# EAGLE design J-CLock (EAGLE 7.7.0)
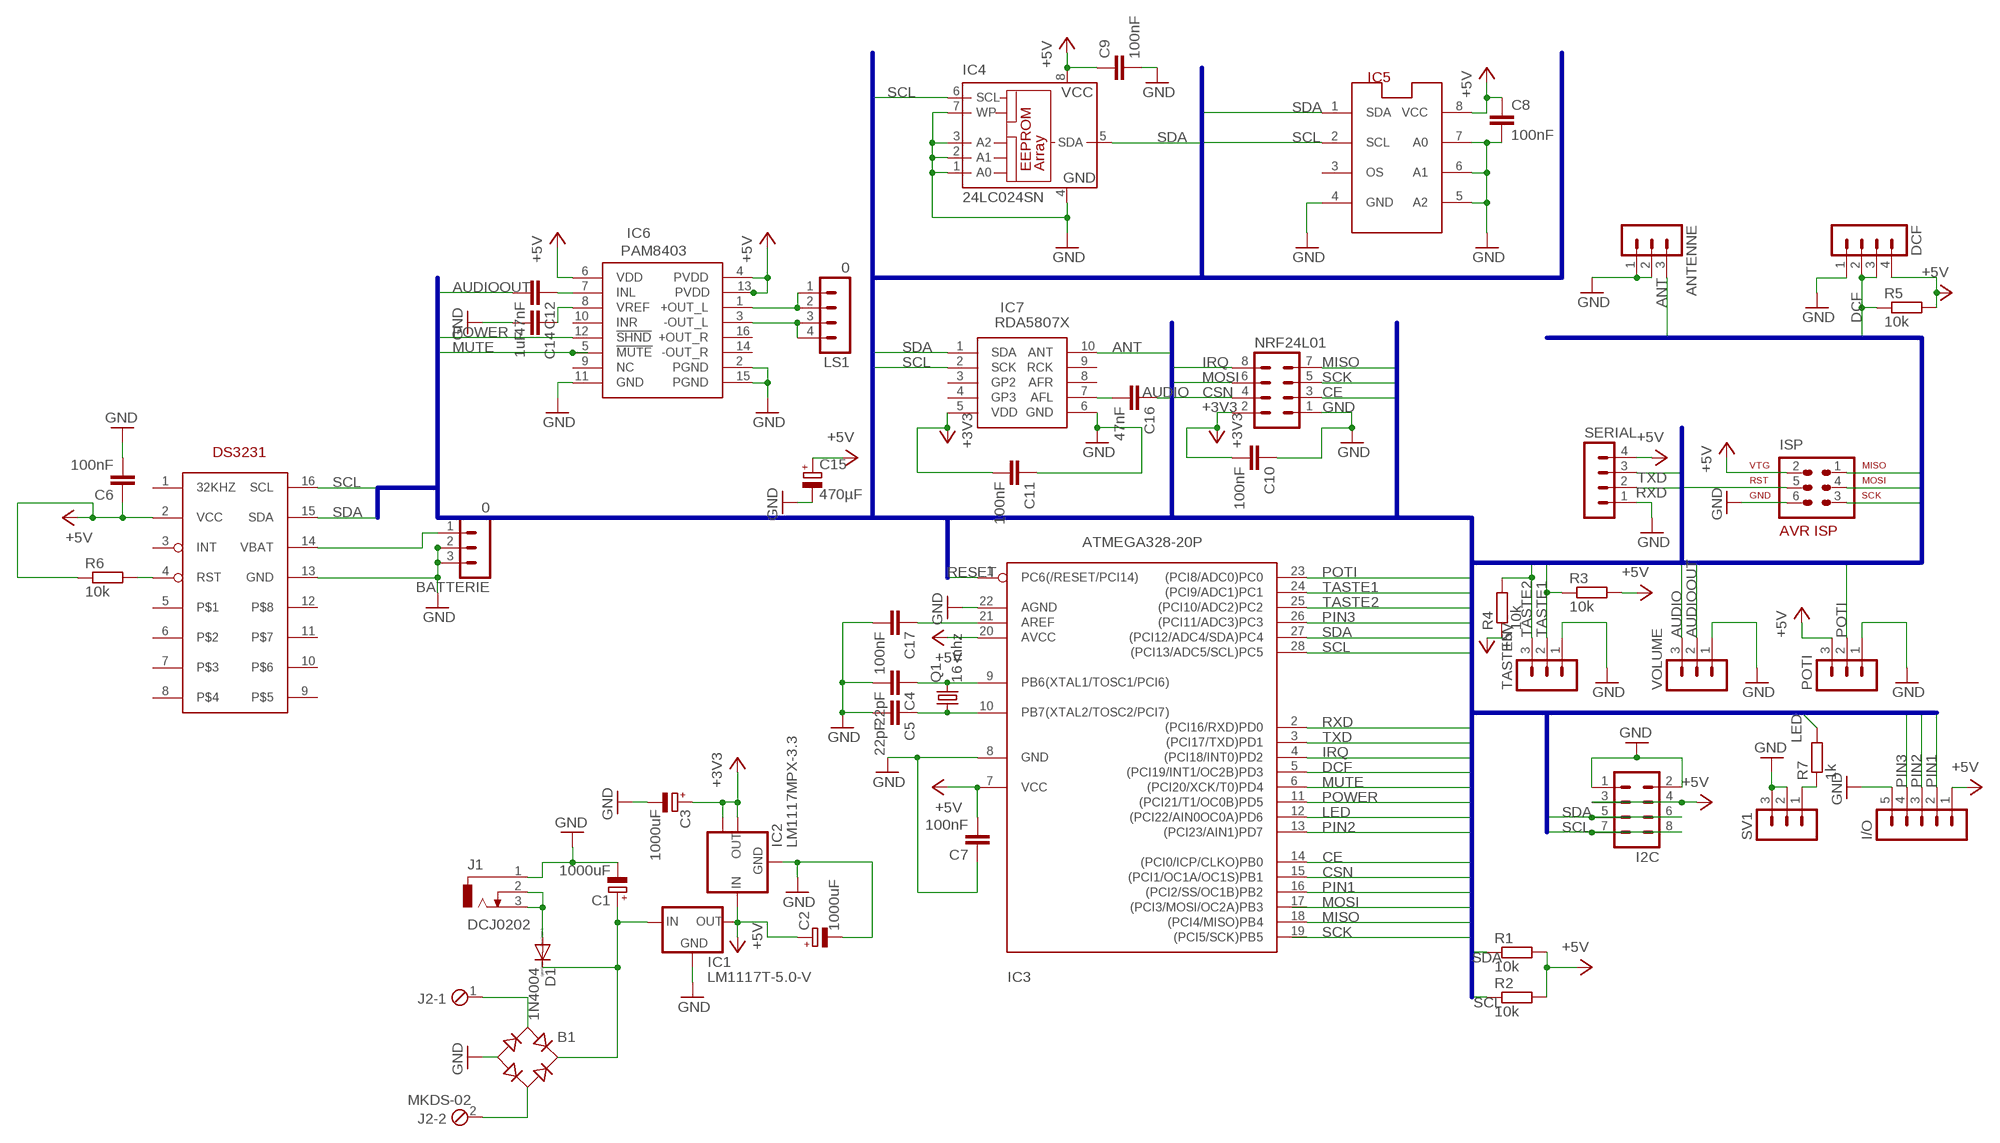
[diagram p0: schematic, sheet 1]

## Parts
ANTENNE  MA03-1  [MA03-1]
B1  B-DIL  [B-DIL]
BATTERIE  0  MA03-1  [MA03-1]
C1  1000uF  CPOL-EUE5-10.5  [E5-10,5]
C2  1000uF  CPOL-EUE5-10.5  [E5-10,5]
C3  1000uF  CPOL-EUE5-10.5  [E5-10,5]
C4  22pF  C-EU050-030X075  [C050-030X075]
C5  22pF  C-EU050-030X075  [C050-030X075]
C6  100nF  C-EU050-030X075  [C050-030X075]
C7  100nF  C-EU050-030X075  [C050-030X075]
C8  100nF  C-EU050-030X075  [C050-030X075]
C9  100nF  C-EU050-030X075  [C050-030X075]
C10  100nF  C-EU050-030X075  [C050-030X075]
C11  100nF  C-EU050-030X075  [C050-030X075]
C12  47nF  C-EU050-030X075  [C050-030X075]
C14  1uF  C-EU050-030X075  [C050-030X075]
C15  470µF  CPOL-EUE3.5-8  [E3,5-8]
C16  47nF  C-EU050-030X075  [C050-030X075]
C17  100nF  C-EU050-030X075  [C050-030X075]
D1  1N4004  [DO41-10]
DCF  MA04-1  [MA04-1]
I2C  MA04-2  [MA04-2]
I/O  MA05-1  [MA05-1]
IC1  LM1117T-5.0-V  [TO220V]
IC2  LM1117MPX-3.3  [SOT223]
IC3  ATMEGA328-20P  [DIL28-3]
IC4  24LC024SN  [SO-08]
IC5  LM75_ICN  [SO8_LM75]
IC6  PAM8403  [SOP16]
IC7  RDA5807X  [MOD5807]
ISP  AVR-ISP-6  [AVR-ISP-6]
J1  DCJ0202  [DCJ0202]
J2  MKDS-02  [MKDS-02]
LS1  0  MA04-1  [MA04-1]
NRF24L01  MA04-2  [MA04-2]
POTI  MA03-1  [MA03-1]
Q1  16 mhz  CRYSTALHC49S  [HC49/S]
R1  10k  R-EU_0207/5V  [0207/5V]
R2  10k  R-EU_0207/5V  [0207/5V]
R3  10k  R-EU_0207/5V  [0207/5V]
R4  10k  R-EU_0207/5V  [0207/5V]
R5  10k  R-EU_0207/5V  [0207/5V]
R6  10k  R-EU_0207/5V  [0207/5V]
R7  1k  R-EU_0207/5V  [0207/5V]
SERIAL  MA04-1  [MA04-1]
SV1  MA03-1  [MA03-1]
TASTEN  MA03-1  [MA03-1]
U$2  DS3231  [SO16]
VOLUME  MA03-1  [MA03-1]

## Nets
+3V3: C3.+ C10.2 C11.2 IC2.2(OUT) IC2.TAB(OUT1) IC7.5(VDD) NRF24L01.2
+5V: C2.+ C6.1 C7.2 C8.1 C9.1 C15.+ DCF.4 I2C.3 I2C.4 I/O.1 IC1.2(OUT) IC2.3(IN) IC3.7(VCC) IC3.20(AVCC) IC4.8(VCC) IC5.8(VCC) IC6.4(PVDD) IC6.6(VDD) IC6.13(PVDD) ISP.2 POTI.3 R1.2 R2.2 R3.2 R4.1 R5.2 R6.1 SERIAL.4 U$2.2(VCC)
ANT: ANTENNE.3 IC7.10(ANT)
AUDIO: C16.1 VOLUME.3
AUDIOOUT: C12.2 VOLUME.2
CE: IC3.14((PCI0/ICP/CLKO)PB0) NRF24L01.3
CSN: IC3.15((PCI1/OC1A/OC1S)PB1) NRF24L01.4
DCF: DCF.2 DCF.3 IC3.5((PCI19/INT1/OC2B)PD3) R5.1
GND: ANTENNE.1 ANTENNE.2 B1.- BATTERIE.2 BATTERIE.3 C1.- C2.- C3.- C4.2 C5.2 C6.2 C7.1 C8.2 C9.2 C10.1 C11.1 C14.2 C15.- C17.2 DCF.1 I2C.1 I2C.2 I/O.5 IC1.1(GND) IC2.1(GND) IC3.8(GND) IC3.22(AGND) IC4.1(A0) IC4.2(A1) IC4.3(A2) IC4.4(GND) IC4.7(WP) IC5.4(GND) IC5.5(A2) IC5.6(A1) IC5.7(A0) IC6.2(PGND) IC6.11(GND) IC6.15(PGND) IC7.6(GND) ISP.6 J1.1 NRF24L01.1 POTI.1 SERIAL.1 SV1.2 SV1.3 TASTEN.1 U$2.13(GND) VOLUME.1
IRQ: IC3.4((PCI18/INT0)PD2) NRF24L01.8
LED: IC3.12((PCI22/AIN0OC0A)PD6) R7.2
MISO: IC3.18((PCI4/MISO)PB4) ISP.1 NRF24L01.7
MOSI: ISP.4 NRF24L01.6
MUTE: IC3.6((PCI20/XCK/T0)PD4) IC6.5(!MUTE!)
N$1: B1.AC2 J2.2
N$2: C4.1 IC3.9(PB6(XTAL1/TOSC1/PCI6)) Q1.2
N$3: B1.+ C1.+ D1.C IC1.3(IN)
N$4: C5.1 IC3.10(PB7(XTAL2/TOSC2/PCI7)) Q1.1
N$5: BATTERIE.1 U$2.14(VBAT)
N$6: D1.A J1.2 J1.3
N$7: B1.AC1 J2.1
N$8: R6.2 U$2.4(RST)
N$9: IC6.1(+OUT_L) LS1.1 LS1.2
N$11: C16.2 IC7.7(AFL)
N$12: C17.1 IC3.21(AREF)
N$14: R7.1 SV1.1
N$16: IC6.3(-OUT_L) LS1.3 LS1.4
N$17: C12.1 IC6.7(INL)
N$18: C14.1 IC6.8(VREF)
PIN1: I/O.2 IC3.16((PCI2/SS/OC1B)PB2)
PIN2: I/O.3 IC3.13((PCI23/AIN1)PD7)
PIN3: I/O.4 IC3.26((PCI11/ADC3)PC3)
POTI: IC3.23((PCI8/ADC0)PC0) POTI.2
POWER: IC3.11((PCI21/T1/OC0B)PD5) IC6.12(!SHND!)
RESET: IC3.1(PC6(/RESET/PCI14)) ISP.5
RXD: IC3.2((PCI16/RXD)PD0) SERIAL.2
SCK: ISP.3 NRF24L01.5
SCL: I2C.7 I2C.8 IC3.28((PCI13/ADC5/SCL)PC5) IC4.6(SCL) IC5.2(SCL) IC7.2(SCK) R2.1 U$2.16(SCL)
SDA: I2C.5 I2C.6 IC3.27((PCI12/ADC4/SDA)PC4) IC4.5(SDA) IC5.1(SDA) IC7.1(SDA) R1.1 U$2.15(SDA)
TASTE1: IC3.24((PCI9/ADC1)PC1) R3.1 TASTEN.2
TASTE2: IC3.25((PCI10/ADC2)PC2) R4.2 TASTEN.3
TXD: IC3.3((PCI17/TXD)PD1) SERIAL.3
Unconnected: IC3.17((PCI3/MOSI/OC2A)PB3) IC3.19((PCI5/SCK)PB5) IC5.3(OS) IC6.9(NC) IC6.10(INR) IC6.14(-OUT_R) IC6.16(+OUT_R) IC7.3(GP2) IC7.4(GP3) IC7.8(AFR) IC7.9(RCK) U$2.1(32KHZ) U$2.3(INT) U$2.5 U$2.6 U$2.7 U$2.8 U$2.9 U$2.10 U$2.11 U$2.12

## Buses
CE,CSN,SCK,MOSI,MISO,IRQ,RESET,SDA,SCL,TXD,RXD,TASTE1,TASTE2,POTI,DCF,MUTE,POWER,LED,AUDIO,AUDIOOUT,LS+,LS-,ANT,PIN1,PIN2,PIN3

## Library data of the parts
ANTENNE BATTERIE POTI SV1 TASTEN VOLUME = con-lstb:MA03-1: PIN HEADER; OC_FARNELL: unknown; OC_NEWARK: unknown
B1 = rectifier:B-DIL: RECTIFIER
C1-C3 C15 = resistor:CPOL-EU: POLARIZED CAPACITOR, European symbol
C4-C12 C14 C16 C17 = resistor:C-EU: CAPACITOR, European symbol
D1 = diode:1N4004: DIODE
DCF LS1 SERIAL = con-lstb:MA04-1: PIN HEADER; OC_FARNELL: unknown; OC_NEWARK: unknown
I2C NRF24L01 = con-lstb:MA04-2: PIN HEADER; OC_FARNELL: unknown; OC_NEWARK: unknown
I/O = con-lstb:MA05-1: PIN HEADER; OC_FARNELL: unknown; OC_NEWARK: unknown
IC1 = lm1117:LM1117T-*
IC2 = lm1117:LM1117MPX-*
IC3 = atmega328:ATMEGA328*P: MICROCONTROLLER 32 kBytes FLASH 2 kBytes SRAM 1 kBytes EEPROM USART 8-channel 10 bit ADC
IC4 = microchip:24*: Serial EEPROM I2C; MF: MICROCHIP; MPN: 24LC024/SN; OC_FARNELL: 1659744; OC_NEWARK: 92C7092
IC5 = lm75:LM75_IC: Temperatursensor
IC6 = RDA5807:PAM8403
IC7 = RDA5807:RDA5807
ISP = avr-6:AVR-ISP-6: AVR ISP-6 Serial Programming Header
J1 = con-jack:DCJ0202: DC POWER JACK Source: DCJ0202.pdf; OC_FARNELL: unknown; OC_NEWARK: unknown
J2 = con-phoenix-500:MKDS-02: MKDSN COMBICON SERIES
Q1 = crystal:CRYSTAL: CRYSTAL; OC_FARNELL: 1667008; OC_NEWARK: unknown
R1-R7 = resistor:R-EU_: RESISTOR, European symbol
U$2 = DS3231:DS3231

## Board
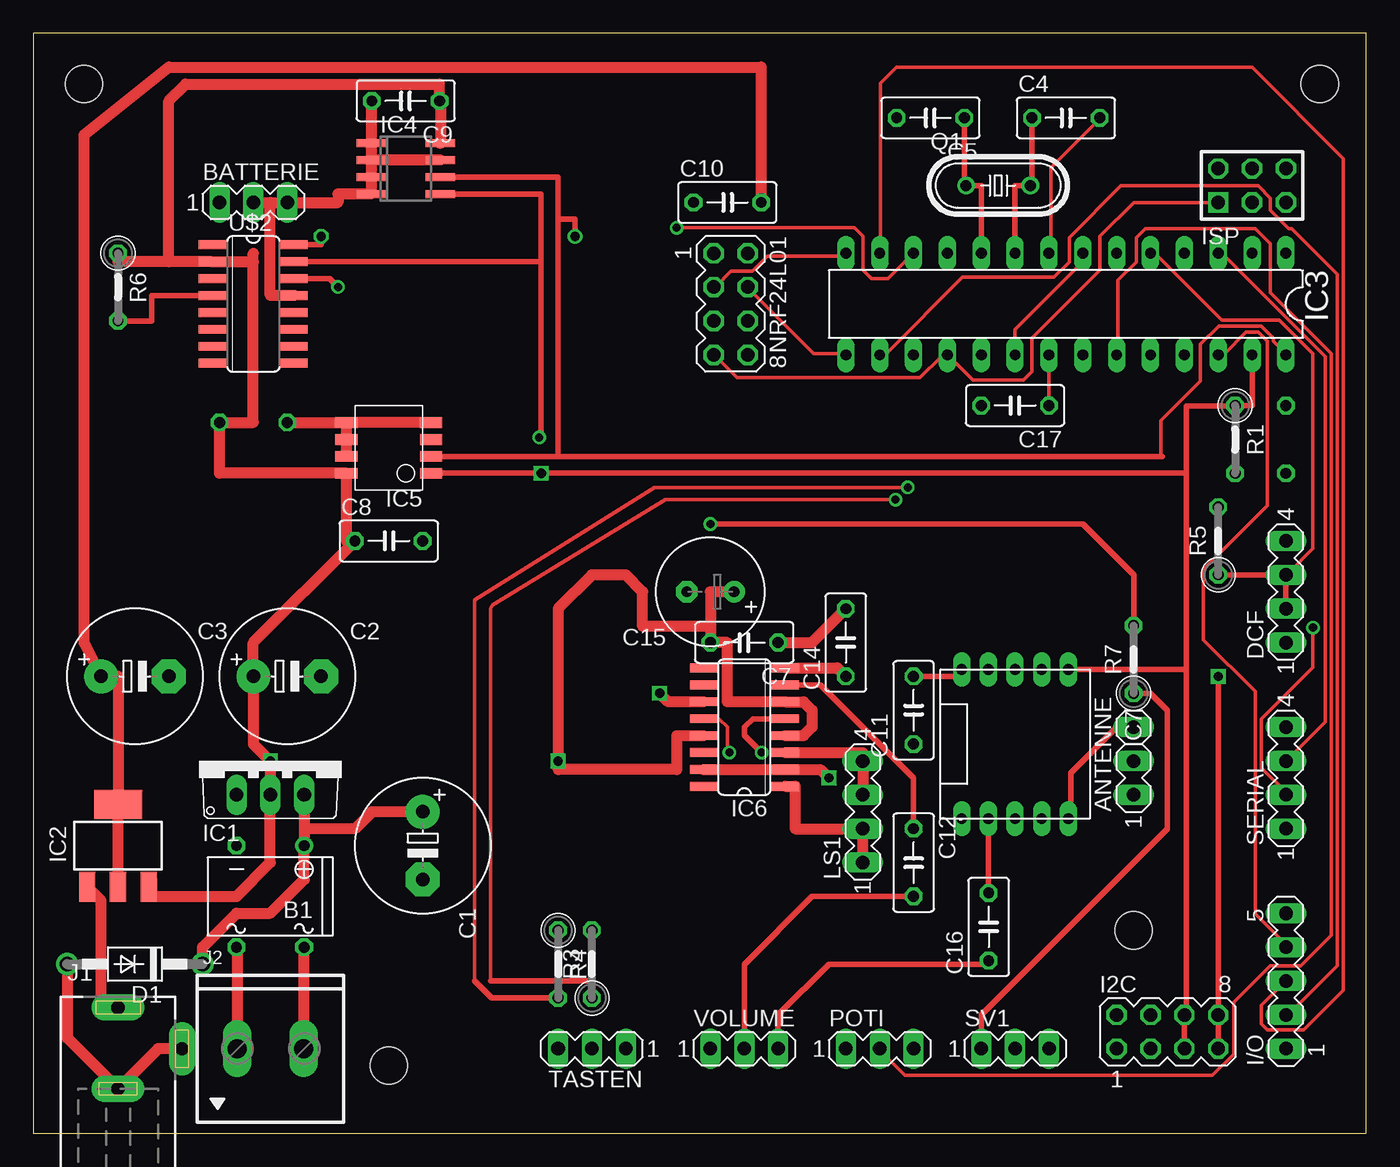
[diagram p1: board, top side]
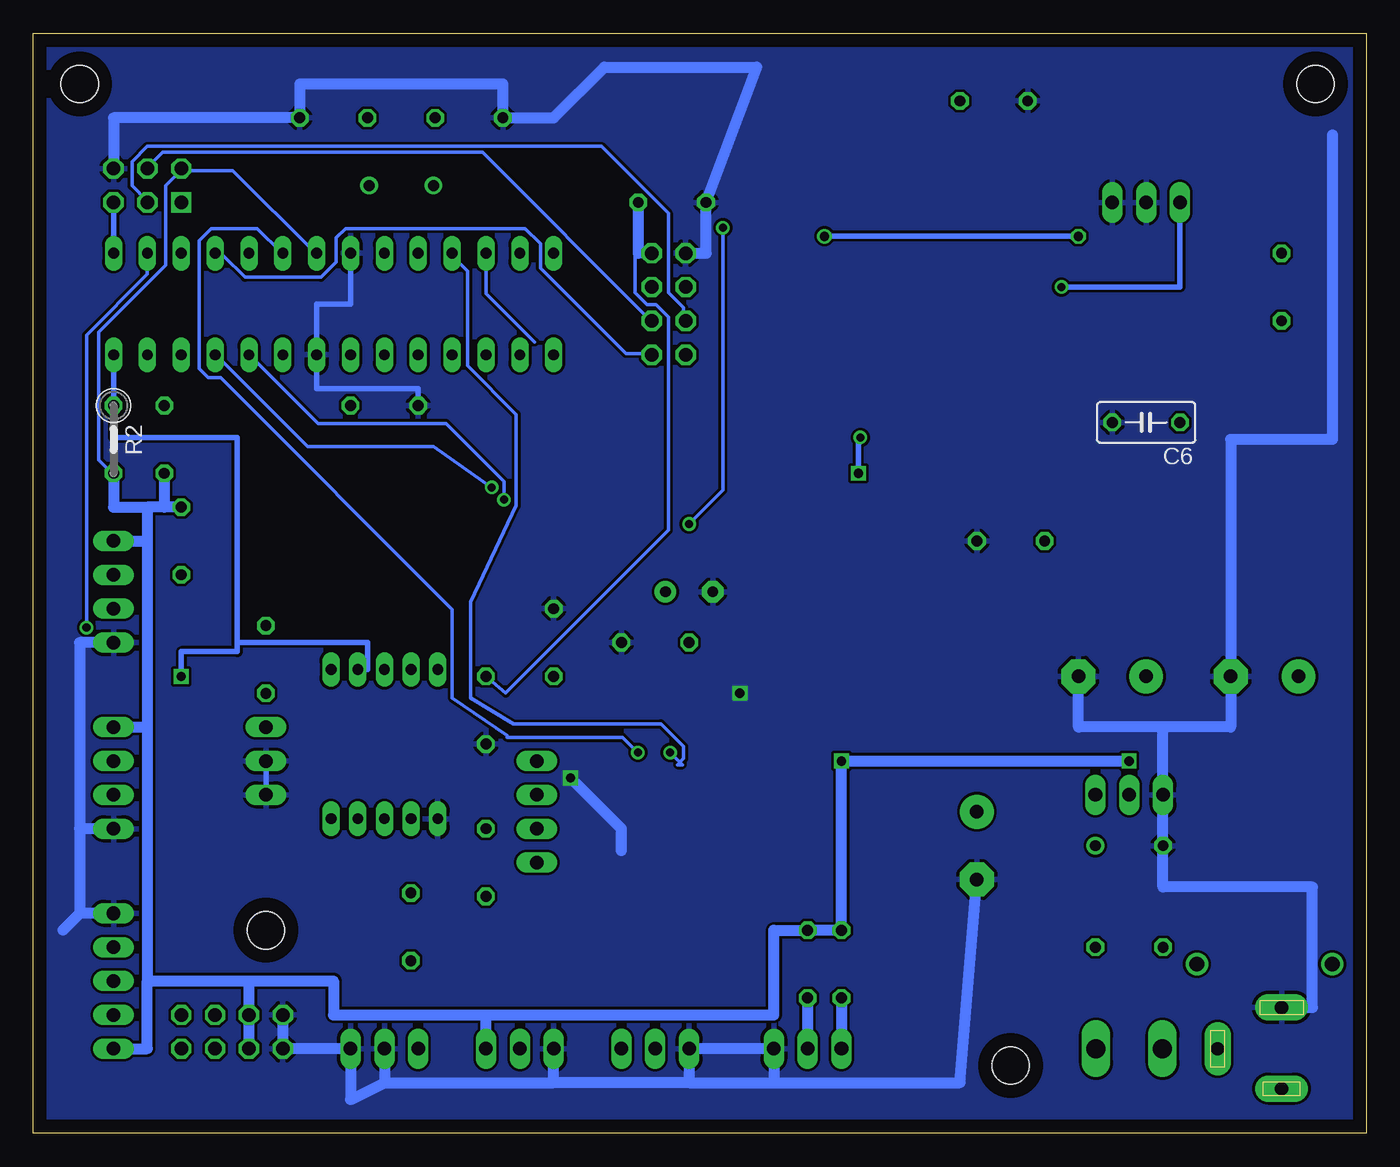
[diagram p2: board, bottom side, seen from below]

Size 100 x 82.54 mm. Coordinates in mm from the lower left corner, seen from the top.
Outline: 0,0 100,0 100,82.54 0,82.54 0,0
Copper layers (1*16): Top 0.035mm / dielectric 1.5mm / Bottom 0.035mm
Design rules "default": minimum track width 10mil, minimum drill 24mil, track to track 8mil, track to pad 8mil, pad to pad 8mil, via to via 8mil, smd to smd 8mil, copper to edge 40mil, drill to drill 8mil, minimum pad ring 10mil, minimum via ring 8mil, stop-mask expansion 4mil, vias tented up to drill 0mil, thermal gap 10mil
Holes 2.8 mm at 82.55,15.24 26.67,5.08 3.81,78.74 96.52,78.74

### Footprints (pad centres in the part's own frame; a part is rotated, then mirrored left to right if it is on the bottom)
MA03-1 = drill 1.016 long: 1 -2.54,0; 2 0,0; 3 2.54,0
B-DIL = drill 0.813: + -2.54,-3.81 | drill 0.813 octagon: - 2.54,-3.81; AC1 2.54,3.81; AC2 -2.54,3.81
E5-10,5 = drill 1.016 pad 2.54: + -2.54,0 | drill 1.016 pad 2.54 octagon: - 2.54,0
C050-030X075 = drill 0.813 octagon: 1 -2.54,0; 2 2.54,0
E3,5-8 = drill 0.813 pad 1.6: + -1.778,0 | drill 0.813 pad 1.6 octagon: - 1.778,0
DO41-10 = drill 1.118: A 5.08,0; C -5.08,0
MA04-1 = drill 1.016 long: 1 -3.81,0; 2 -1.27,0; 3 1.27,0; 4 3.81,0
MA04-2 = drill 1.016 octagon: 1 -3.81,-1.27; 2 -3.81,1.27; 3 -1.27,-1.27; 4 -1.27,1.27; 5 1.27,-1.27; 6 1.27,1.27; 7 3.81,-1.27; 8 3.81,1.27
MA05-1 = drill 1.016 long: 1 -5.08,0; 2 -2.54,0; 3 0,0; 4 2.54,0; 5 5.08,0
TO220V = drill 1.016 long: 1 -2.54,-2.54; 2 0,-2.54; 3 2.54,-2.54
SOT223 = smd 1.219 x 2.235: 1 -2.311,-3.099; 2 0,-3.099; 3 2.311,-3.099 | smd 3.6 x 2.2: TAB 0,3.099
DIL28-3 = drill 0.813 long: 1 -16.51,-3.81; 2 -13.97,-3.81; 3 -11.43,-3.81; 4 -8.89,-3.81; 5 -6.35,-3.81; 6 -3.81,-3.81; 7 -1.27,-3.81; 8 1.27,-3.81; 9 3.81,-3.81; 10 6.35,-3.81; 11 8.89,-3.81; 12 11.43,-3.81; 13 13.97,-3.81; 14 16.51,-3.81; 15 16.51,3.81; 16 13.97,3.81; 17 11.43,3.81; 18 8.89,3.81; 19 6.35,3.81; 20 3.81,3.81; 21 1.27,3.81; 22 -1.27,3.81; 23 -3.81,3.81; 24 -6.35,3.81; 25 -8.89,3.81; 26 -11.43,3.81; 27 -13.97,3.81; 28 -16.51,3.81
SO-08 = smd 0.6 x 2.2: 1 -1.905,-2.6; 2 -0.635,-2.6; 3 0.635,-2.6; 4 1.905,-2.6; 5 1.905,2.6; 6 0.635,2.6; 7 -0.635,2.6; 8 -1.905,2.6
SO8_LM75 = smd 0.813 x 1.676: 1 -1.27,-3.175; 2 0,-3.175; 3 1.27,-3.175; 4 2.54,-3.175; 5 2.54,3.175; 6 1.27,3.175; 7 0,3.175; 8 -1.27,3.175
SOP16 = smd 0.66 x 2.032: 1 -4.445,-3.073; 2 -3.175,-3.073; 3 -1.905,-3.073; 4 -0.635,-3.073; 5 0.635,-3.073; 6 1.905,-3.073; 7 3.175,-3.073; 8 4.445,-3.073; 9 4.445,3.073; 10 3.175,3.073; 11 1.905,3.073; 12 0.635,3.073; 13 -0.635,3.073; 14 -1.905,3.073; 15 -3.175,3.073; 16 -4.445,3.073
MOD5807 = drill 0.8 pad 1.27 long: 1 -5.6,4; 2 -5.6,2; 3 -5.6,0; 4 -5.6,-2; 5 -5.6,-4; 6 5.6,-4; 7 5.6,-2; 8 5.6,0; 9 5.6,2; 10 5.6,4
AVR-ISP-6 = drill 1.016 square: 1 -2.54,-1.27 | drill 1.016 octagon: 2 -2.54,1.27; 3 0,-1.27; 4 0,1.27; 5 2.54,-1.27; 6 2.54,1.27
DCJ0202 = drill 1 pad 2 long: 1 0,3.1; 2 4.8,0; 3 0,-3
MKDS-02 = drill 1.422 long: 1 -2.5,0; 2 2.5,0
HC49/S = drill 0.813: 1 -2.413,0; 2 2.413,0
0207/5V = drill 0.813 octagon: 1 -2.54,0; 2 2.54,0
SO16 = smd 0.66 x 2.032: 1 -4.445,-3.073; 2 -3.175,-3.073; 3 -1.905,-3.073; 4 -0.635,-3.073; 5 0.635,-3.073; 6 1.905,-3.073; 7 3.175,-3.073; 8 4.445,-3.073; 9 4.445,3.073; 10 3.175,3.073; 11 1.905,3.073; 12 0.635,3.073; 13 -0.635,3.073; 14 -1.905,3.073; 15 -3.175,3.073; 16 -4.445,3.073

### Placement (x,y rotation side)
ANTENNE  82.55,27.94 90 top
B1  17.78,17.78 180 top
BATTERIE  16.51,69.85 0 top
C1  29.21,21.59 270 top
C2  19.05,34.29 0 top
C3  7.62,34.29 0 top
C4  77.47,76.2 0 top
C5  67.31,76.2 180 top
C6  16.51,53.34 180 bottom
C7  53.34,36.83 180 top
C8  26.67,44.45 0 top
C9  27.94,77.47 180 top
C10  52.07,69.85 0 top
C11  66.04,31.75 90 top
C12  66.04,20.32 270 top
C14  60.96,36.83 90 top
C15  50.8,40.64 180 top
C16  71.68,15.49 90 top
C17  73.66,54.61 180 top
D1  7.62,12.7 180 top
DCF  93.98,40.64 90 top
I2C  85.09,7.62 0 top
I/O  93.98,11.43 90 top
IC1  17.78,27.94 0 top
IC2  6.35,21.59 0 top
IC3  77.47,62.23 180 top
IC4  27.94,72.39 270 top
IC5  26.67,50.8 90 top
IC6  53.34,30.48 90 top
IC7  73.66,29.21 270 top
ISP  91.44,71.12 0 top
J1  6.35,6.35 0 top
J2  17.78,6.35 0 top
LS1  62.23,24.13 90 top
NRF24L01  52.32,62.23 270 top
POTI  63.5,6.35 0 top
Q1  72.39,71.12 0 top
R1  90.17,52.07 270 top
R2  93.98,52.07 270 bottom
R3  41.91,12.7 90 top
R4  39.37,12.7 270 top
R5  88.9,44.45 90 top
R6  6.35,63.5 270 top
R7  82.55,35.56 90 top
SERIAL  93.98,26.67 90 top
SV1  73.66,6.35 0 top
TASTEN  41.91,6.35 180 top
U$2  16.51,62.23 270 top
VOLUME  53.34,6.35 0 top

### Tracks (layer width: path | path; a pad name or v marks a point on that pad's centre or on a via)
+3V3
  Top 0.254: IC7.5 69.85,34.29 69.85,34.28
  Top 0.406: C11.2 65.86,34.29 65.86,34.28 69.85,34.28
  Top 0.813: IC2.2 IC2.TAB 6.35,34.29 C3.+ 3.81,36.83 3.81,74.93 10.16,80.01 54.61,80.01 C10.2
  Bottom 0.254: NRF24L01.2 53.72,66.06 53.72,66.04 | 54.61,66.04 54.86,65.84 54.86,63.09 53.95,62.18 53.26,62.18 52.35,61.27 52.35,45.26 64.57,33.05 C11.2
  Bottom 0.813: 53.34,66.04 NRF24L01.2 53.72,66.04 54.61,66.04 C10.2
+5V  (via drill 0.7)
  Top 0.254: 50.98,40.69 50.8,40.64 | 52.58,40.69 C15.+ | IC3.20 73.66,60.33 78.74,65.41 IC3.7
  Top 0.813: IC2.3 8.66,19.05 8.89,19.05 8.89,17.78 15.24,17.78 17.78,20.32 IC1.2 v17.78,27.94 16.51,29.21 C2.+ 16.51,36.83 C8.1 23.5,44.45 IC5.8 13.97,49.53 C6.1 16.51,53.34 16.51,65.41 | 50.8,38.05 50.8,40.64 C15.+ | 50.8,38.05 C7.2 52.07,36.83 52.07,32.38 IC6.6 57.78,32.38 58.42,31.75 58.42,30.48 57.78,29.84 IC6.4 | 16.51,65.41 16.51,66.04 | 16.51,65.41 U$2.2 10.16,65.41 | IC4.8 30.54,77.47 C9.1 30.48,78.74 11.43,78.74 10.16,77.47 10.16,65.41 | 10.16,65.41 6.35,65.41 R6.1 | 50.8,38.05 45.72,38.05 45.72,40.64 44.45,41.91 41.91,41.91 39.37,39.37 v39.37,27.94 39.37,27.3 48.26,27.3 48.26,29.84 IC6.13
  Bottom 0.254: IC3.7 78.87,66.06 85.04,72.24 88.7,72.24 ISP.2 88.92,72.24 90.07,71.09 90.07,65.15 95.1,60.12 95.1,50.52 94.18,49.61 R2.2
  Bottom 0.813: v17.78,27.94 v39.37,27.94 R4.1 R3.2 44.45,15.24 44.45,8.89 66.04,8.89 | POTI.3 66.04,8.89 | I2C.3 I2C.4 83.82,11.43 | 83.82,11.43 77.47,11.43 77.47,8.89 66.04,8.89 | I/O.1 91.44,6.35 91.44,11.43 | 91.44,11.43 83.82,11.43 | SERIAL.4 91.44,30.48 | 91.44,30.48 91.44,11.43 | DCF.4 91.44,44.45 | 91.44,44.45 91.44,30.48 | R5.2 90.17,46.99 | 90.17,46.99 91.44,46.99 | 91.44,46.99 91.44,44.45 | R2.2 93.98,46.99 91.44,46.99 | R1.2 90.17,46.99
ANT
  Top 0.406: ANTENNE.3 81.28,30.48 77.85,27.05 77.85,23.61 IC7.10
AUDIO
  Top 0.406: VOLUME.3 55.88,8.89 59.69,12.7 71.42,12.7 C16.1
AUDIOOUT
  Top 0.406: VOLUME.2 53.34,12.7 58.42,17.78 C12.2
CE
  Top 0.254: IC3.14 60.81,65.84 55.09,65.84 53.95,64.69 52.35,64.69 51.21,63.55 NRF24L01.3
CSN
  Top 0.254: IC3.15 60.81,58.52 58.52,58.52 53.72,63.32 NRF24L01.4
DCF
  Top 0.254: IC3.5 83.9,65.84 84.35,65.84 89.15,61.04 93.5,61.04 96.01,58.52 96.01,43.89 94.18,42.06 DCF.3
  Top 0.406: DCF.2 DCF.3 R5.1
GND  (via drill 0.7)
  Top 0.254: 4.12,18.29 IC2.1 | IC3.8 76.35,66.06 76.35,72.47 80.01,76.12 C4.2
  Top 0.813: IC5.7 IC5.6 IC5.5 | C6.2 IC5.5 | U$2.13 17.78,62.87 17.78,69.85 | 17.78,69.85 BATTERIE.3 22.86,69.85 22.86,70.48 IC4.4 IC4.3 IC4.2 | C9.2 25.34,77.47 IC4.1 IC4.2 | BATTERIE.2 17.78,69.85 | IC4.7 IC4.2 | J1.1 5.79,9.45 5.08,10.16 5.08,17.45 IC2.1 | IC5.4 IC5.5 | IC6.15 IC6.2 59.05,27.3 v59.69,26.67 | IC6.11 47.62,32.38 v46.99,33.02 | C7.1 58.42,36.83 C14.2
  Bottom 0.254: NRF24L01.1 50.98,66.06 50.8,66.04
  Bottom 0.406: IC3.8 76.2,62.23 78.74,62.23 IC3.22 78.74,55.88 71.12,55.88 C17.2 | ANTENNE.2 ANTENNE.1
  Bottom 0.813: J1.1 4.04,9.45 IC2.1 15.24,18.49 B1.- IC1.1 15.24,30.48 | 15.24,30.48 21.59,30.48 C2.- | 15.24,30.48 10.16,30.48 C3.- 10.16,52.07 2.54,52.07 2.54,74.93 | 44.45,3.81 TASTEN.1 VOLUME.1 50.8,3.81 | 44.45,3.81 30.48,3.81 C1.- | 50.8,3.81 60.96,3.81 | 60.96,3.81 POTI.1 | SV1.2 73.66,3.81 | 73.66,3.81 60.96,3.81 | 73.66,3.81 76.2,2.54 SV1.3 I2C.1 I2C.2 | I/O.5 96.52,16.51 | SERIAL.1 96.52,22.86 | 96.52,22.86 96.52,16.51 | DCF.1 96.52,36.83 96.52,22.86 | 50.8,3.81 44.45,3.81 | ISP.6 93.98,76.2 C4.2 80.01,78.74 64.77,78.74 C5.2 60.96,76.2 57.15,80.01 45.72,80.01 C10.1 49.53,66.04 50.8,66.04 | 97.79,15.24 96.52,16.51 | 55.88,21.23 55.88,22.86 v59.69,26.67
  pour Bottom: 100.33,82.55 0,82.55 0,0 100.33,0
IRQ
  Bottom 0.254: IC3.4 86.18,65.84 85.72,65.84 84.12,64.24 78.41,64.24 77.27,65.38 77.27,67.21 76.58,67.89 63.09,67.89 61.95,66.75 61.95,64.92 55.55,58.52 53.72,58.52 NRF24L01.8
LED  (via drill 0.61)
  Top 0.254: IC3.12 64.14,64.14 62.87,64.14 62.23,64.77 62.23,67.31 61.59,67.94 v48.26,67.94
  Top 0.406: R7.2 82.55,41.91 78.74,45.72 v50.8,45.72
  Bottom 0.254: IC3.12 66.04,63.02 62.39,59.37 | v48.26,67.94 48.26,48.26 v50.8,45.72
MISO
  Top 0.254: NRF24L01.7 51.21,58.29 52.81,56.69 66.52,56.69 68.12,58.29 68.58,58.29 IC3.18 70.48,56.52 74.3,56.52 74.93,57.15 74.93,59.69 80.01,64.77 80.01,67.31 82.55,69.85 ISP.1
MOSI
  Bottom 0.254: NRF24L01.6 53.72,61.04 66.29,73.61 90.3,73.61 91.44,72.47 ISP.4
MUTE  (via drill 0.61)
  Top 0.406: IC6.5 53.98,31.11 53.34,30.48 53.34,29.87 v54.63,28.57
  Bottom 0.254: IC3.6 81.38,66.06 83.21,67.89 86.64,67.89 87.55,66.98 87.55,57.38 86.87,56.69 85.95,56.69 68.58,39.32 68.58,32.69 64.47,29.84 64.47,29.72 55.8,29.72 54.66,28.57 v54.63,28.57
N$1
  Top 0.813: B1.AC2 20.28,13.97 J2.2
N$2
  Top 0.406: IC3.9 73.66,71.12 Q1.2 74.93,71.12 C4.1
N$3
  Top 0.813: IC1.3 20.32,22.86 | 20.32,22.86 B1.+ 20.32,19.05 17.78,16.51 15.24,16.51 12.7,13.97 D1.C | C1.+ 25.4,24.13 24.13,22.86 20.32,22.86
N$4
  Top 0.406: IC3.10 71.12,71.12 Q1.1 69.85,71.12 C5.1
N$5  (via drill 0.61)
  Top 0.406: U$2.14 22.23,64.14 v22.86,63.5
  Bottom 0.406: BATTERIE.1 13.97,63.5 v22.86,63.5
N$6
  Top 0.813: J1.2 9.35,6.35 J1.3 2.54,7.16 D1.A
N$7
  Top 0.813: B1.AC1 15.28,13.97 J2.1
N$8
  Top 0.406: U$2.4 8.89,62.87 8.89,60.96 R6.2
N$9
  Top 0.813: IC6.1 57.15,26.04 57.15,22.86 LS1.2 LS1.1
N$11
  Top 0.406: C16.2 71.66,18.49 IC7.7
N$12
  Top 0.254: IC3.21 C17.1
N$14
  Top 0.406: SV1.1 71.12,8.89 85.09,22.86 85.09,31.75 83.82,33.02 R7.1
N$16
  Top 0.813: IC6.3 62.23,28.57 LS1.4 LS1.3
N$17
  Top 0.406: C12.1 66.04,26.67 59.05,33.66 IC6.7
N$18
  Top 0.813: IC6.8 60.33,34.92 C14.1
PIN1
  Top 0.254: IC3.16 63.55,58.52 64.01,58.52 69.72,64.24 76.58,64.24 77.72,65.38 77.72,67.21 81.61,71.09 91.9,71.09 92.81,70.18 92.81,69.27 94.18,67.89 94.41,67.89 97.84,64.47 97.84,12.57 94.18,8.91 I/O.2
PIN2
  Top 0.254: IC3.13 63.55,66.06 63.55,78.79 64.77,80.01 91.44,80.01 98.3,73.15 98.3,10.74 95.33,7.77 92.58,7.77 92.13,8.23 92.13,9.6 93.95,11.43 I/O.3
PIN3
  Top 0.254: IC3.26 88.92,58.52 89.38,58.52 90.98,60.12 91.9,60.12 92.58,59.44 92.58,47.09 87.78,42.29 87.78,37.03 91.67,33.15 91.67,16.46 93.95,14.17 I/O.4
POTI
  Top 0.254: IC3.23 81.38,58.52 81.38,64.01 82.75,65.38 82.75,67.21 83.44,67.89 91.67,67.89 92.81,66.75 92.81,63.09 97.38,58.52 97.38,14.86 95.1,12.57 92.81,12.57 90.07,9.83 90.07,5.94 88.47,4.34 65.38,4.34 63.55,6.17 POTI.2
POWER  (via drill 0.61)
  Top 0.254: IC6.12 51.44,31.11 52.07,30.48 52.07,28.57 v52.22,28.57
  Bottom 0.254: v52.22,28.57 51.31,27.66 51.66,27.66 51.21,28.12 51.21,29.03 52.91,30.73 63.98,30.73 67.21,32.69 67.21,39.85 63.78,47.09 63.78,53.95 67.44,57.61 67.44,64.69 68.58,65.84 IC3.11
RESET
  Bottom 0.406: ISP.5 IC3.1
RXD  (via drill 0.61)
  Top 0.254: v96.01,37.95 96.01,34.98 92.13,31.09 92.13,27.43 93.95,25.6 SERIAL.2
  Bottom 0.254: IC3.2 91.44,64.47 96.01,59.89 v96.01,37.95
SCK
  Bottom 0.254: NRF24L01.5 51.21,61.04 51.21,61.95 52.35,63.09 52.35,69.04 57.38,74.07 91.44,74.07 92.58,72.92 92.58,71.09 91.44,69.95 ISP.3
SCL  (via drill 0.7, 0.7 pad 0.41)
  Top 0.254: 84.58,50.8 84.58,53.49 87.55,56.46 87.55,59.21 88.92,60.58 92.13,60.58 93.04,59.66 93.04,59.44 93.95,58.52 IC3.28
  Top 0.406: I2C.7 I2C.8 v88.9,34.29 | IC5.2 39.37,50.8 | 39.37,50.8 84.58,50.8 84.7,50.8 | 39.37,68.58 39.37,71.75 IC4.6 | 39.37,68.58 39.37,50.8 | U$2.16 21.59,66.67 v21.59,67.31 | v40.64,67.31 40.64,68.58 39.37,68.58
  Bottom 0.406: IC3.28 R2.1 93.98,52.22 84.7,52.22 84.7,36.83 | 84.7,36.83 84.7,36.14 88.9,36.14 v88.9,34.29 | v21.59,67.31 v40.64,67.31 | IC7.2 74.93,34.81 74.93,36.83 84.7,36.83
SDA  (via drill 0.61, 0.7)
  Top 0.254: 38.1,52.35 37.95,52.35 v37.95,52.22
  Top 0.406: IC3.27 91.44,54.61 R1.1 90.17,54.59 86.5,54.59 86.5,49.53 | I2C.5 I2C.6 86.5,8.89 86.5,34.81 | 86.5,34.81 86.5,49.53 | IC5.1 v38.1,49.53 86.5,49.53 | 38.1,65.41 38.1,70.48 IC4.5 | 38.1,65.41 38.1,52.35 38.1,52.07 | U$2.15 38.1,65.41 | IC7.1 86.5,34.81
  Bottom 0.406: v38.1,49.53 38.1,52.07 v37.95,52.22
TASTE1  (via drill 0.61)
  Top 0.254: v64.69,47.55 47.42,47.55 34.44,39.65 34.49,39.65 34.39,39.55 34.29,39.37 34.29,11.43
  Top 0.406: R3.1 41.91,11.43 34.29,11.43
  Bottom 0.254: v64.69,47.55 64.69,48.92 69.04,53.26 78.64,53.26 83.67,58.29 IC3.24
  Bottom 0.813: R3.1 TASTEN.2
TASTE2  (via drill 0.61)
  Top 0.254: v65.61,48.46 46.61,48.46 33.1,40.03 33.1,11.43 | 39.32,10.29 R4.2
  Top 0.406: R4.2 34.37,10.16 33.1,11.43
  Bottom 0.254: v65.61,48.46 69.95,51.54 79.43,51.54 86.18,58.29 IC3.25
  Bottom 0.813: R4.2 TASTEN.3
TXD
  Top 0.254: IC3.3 88.92,65.84 89.38,65.84 96.93,58.29 96.93,30.86 94.18,28.12 SERIAL.3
